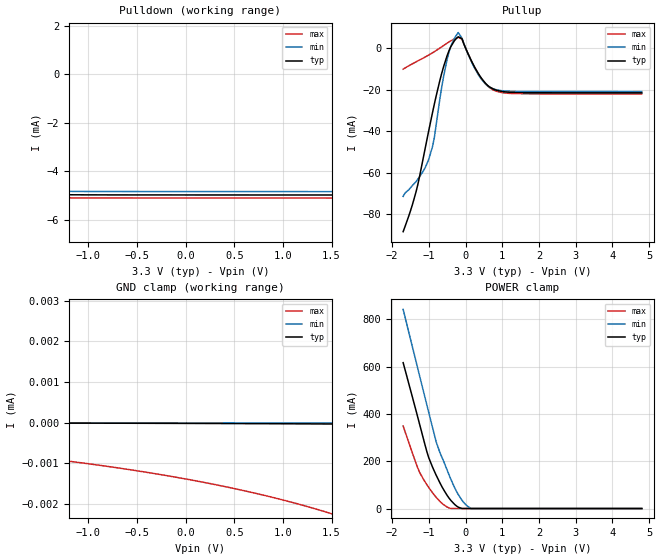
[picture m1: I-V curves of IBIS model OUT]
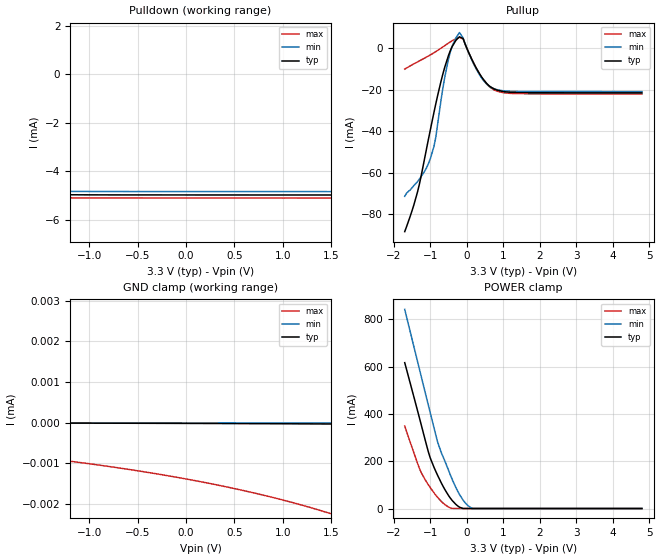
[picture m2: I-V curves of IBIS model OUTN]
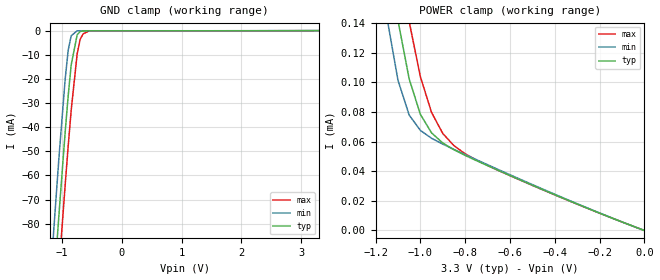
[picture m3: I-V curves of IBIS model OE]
| IBIS File ea2102.ibs
[IBIS Ver]   3.2
[File name]   ea2102.ibs
[File Rev]   1.1
[Date]   April 07,2008
[Disclaimer]
Epson Toyocom Corporation makes no warranty with respect to the information
contained herein.
[Copyright]
Copyright(C) 2008, Epson Toyocom Corporation. All rights reserved.
|   Component EA-2102CB
[Component]   EA-2102CB
Si_location Pin
Timing_location Pin
[Manufacturer]   Epson Toyocom Corporation
[Package]
| variable   typ   min   max
R_pkg   1.04   NA   NA
L_pkg   1.98n   NA   NA
C_pkg   3.71p   NA   NA
[Pin] signal_name   model_name
1   OE   OE
3   GND   GND
4   OUT   OUT
5   OUTN   OUTN
6   VCC   POWER
| Models and submodels in the file (3): OUT (3-state_ECL), OUTN (3-state_ECL), OE (Input)
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|   Model OUT
[Model]   OUT
Model_type 3-state_ECL
Enable Active-High
Polarity Non-Inverting
Vref=1.3
Vmeas=1.97
Rref=50
C_comp   3p   NA   NA
[Temperature Range] 25   -40   85
[Voltage Range]   3.3   3   3.6
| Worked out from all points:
|   GND clamp passes 1 mA (typ) near -3.42 V on its own axis
|   POWER clamp passes 1 mA (typ) near -0.12 V on its own axis
[Pullup]
-1.7V     -88.4mA    -71.42mA   -10.14mA
-1.35V    -69.31mA   -64.36mA   -6.662mA
-1V       -39.54mA   -53.37mA   -3.319mA
-850mV    -26.97mA   -43.09mA   -1.734mA
-650mV    -12.19mA   -18.88mA   598.7uA
-500mV    -3.531mA   -5.232mA   2.399mA
-400mV    718.1uA    1.011mA    3.511mA
-200mV    5.42mA     7.472mA    5.095mA
-100mV    4.565mA    4.85mA     4.38mA
350mV     -12.37mA   -12.87mA   -12.43mA
800mV     -20.07mA   -19.88mA   -20.56mA
4.8V      -21.56mA   -20.96mA   -22.11mA
[Pulldown]
-5V       -23.85mA   -20.89mA   -6.093mA
-4.35V    -14.27mA   -18.44mA   -4.063mA
-3.95V    -6.468mA   -15.25mA   -1.174mA
-3.75V    -3.048mA   -10.1mA    1.119mA
-3.7V     -2.251mA   -8.541mA   1.051mA
-3.6V     -714.4uA   -5.714mA   -1.09nA
-3.5V     888.6uA    -3.303mA   -953.3uA
-3.4V     1.098mA    -1.336mA   -1.821mA
-3.15V    -1.401mA   1.865mA    -3.569mA
-2.7V     -4.216mA   -2.707mA   -4.892mA
-2.25V    -4.871mA   -4.555mA   -5.062mA
1.5V      -4.978mA   -4.838mA   -5.103mA
[GND Clamp]
-5V       616.4mA    841.5mA    348.7mA
-3.7V     34.04mA    123.3mA    185.8uA
-3.6V     17.65mA    88.89mA    326.2fA
-3.55V    11.15mA    73.48mA    -342.5nA
-3.4V     15.09uA    35.4mA     -436.6nA
-3.35V    73.91nA    25.63mA    -447.3nA
-3.3V     0A         17.29mA    -457.5nA
-3.15V    -5.195nA   189.1uA    -487.1nA
-3.1V     -5.365nA   95.47nA    -496.9nA
-3.05V    -5.521nA   147.6pA    -506.6nA
-400mV    -16.4nA    -28.83pA   -1.224uA
1.5V      -33.73nA   -58.18pA   -2.243uA
[POWER Clamp]
-1.7V     616.4mA    841.5mA    348.7mA
-1.35V    414.1mA    622mA      191.6mA
-1.25V    355.1mA    559.5mA    152.4mA
-1.05V    238mA      435.1mA    99.88mA
-900mV    175.1mA    342.6mA    66.68mA
-800mV    140.6mA    281.5mA    47.18mA
-700mV    108.9mA    237mA      30.3mA
-400mV    34.04mA    123.3mA    185.8uA
-200mV    5.735mA    59.39mA    -406.9nA
50mV      -4.322nA   10.2mA     -467.5nA
200mV     -5.365nA   95.47nA    -496.9nA
4.8V      -33.73nA   -58.18pA   -2.243uA
[Ramp]
R_load=50
dV/dt_r   4.714E-1/5.411E-11   4.388E-1/5.767E-11   4.955E-1/5.468E-11
dV/dt_f   4.740E-1/5.706E-11   4.381E-1/6.433E-11   5.010E-1/5.109E-11
| End [model] OUT
|   Model OUTN
[Model]   OUTN
Model_type 3-state_ECL
Enable Active-High
Polarity Inverting
Vref=1.3
Vmeas=1.97
Rref=50
C_comp   3p   NA   NA
[Temperature Range] 25   -40   85
[Voltage Range]   3.3   3   3.6
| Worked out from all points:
|   GND clamp passes 1 mA (typ) near -3.42 V on its own axis
|   POWER clamp passes 1 mA (typ) near -0.12 V on its own axis
[Pullup]
-1.7V     -88.4mA    -71.42mA   -10.14mA
-1.35V    -69.31mA   -64.36mA   -6.662mA
-1V       -39.54mA   -53.37mA   -3.319mA
-850mV    -26.97mA   -43.09mA   -1.734mA
-650mV    -12.19mA   -18.88mA   598.7uA
-500mV    -3.531mA   -5.232mA   2.399mA
-400mV    718.1uA    1.011mA    3.511mA
-200mV    5.42mA     7.472mA    5.095mA
-100mV    4.565mA    4.85mA     4.38mA
350mV     -12.37mA   -12.87mA   -12.43mA
800mV     -20.07mA   -19.88mA   -20.56mA
4.8V      -21.56mA   -20.96mA   -22.11mA
[Pulldown]
-5V       -23.85mA   -20.89mA   -6.093mA
-4.35V    -14.27mA   -18.44mA   -4.063mA
-3.95V    -6.468mA   -15.25mA   -1.174mA
-3.75V    -3.048mA   -10.1mA    1.119mA
-3.7V     -2.251mA   -8.541mA   1.051mA
-3.6V     -714.4uA   -5.714mA   -1.09nA
-3.5V     888.6uA    -3.303mA   -953.3uA
-3.4V     1.098mA    -1.336mA   -1.821mA
-3.15V    -1.401mA   1.865mA    -3.569mA
-2.7V     -4.216mA   -2.707mA   -4.892mA
-2.25V    -4.871mA   -4.555mA   -5.062mA
1.5V      -4.978mA   -4.838mA   -5.103mA
[GND Clamp]
-5V       616.4mA    841.5mA    348.7mA
-3.7V     34.04mA    123.3mA    185.8uA
-3.6V     17.65mA    88.89mA    326.2fA
-3.55V    11.15mA    73.48mA    -342.5nA
-3.4V     15.09uA    35.4mA     -436.6nA
-3.35V    73.91nA    25.63mA    -447.3nA
-3.3V     0A         17.29mA    -457.5nA
-3.15V    -5.195nA   189.1uA    -487.1nA
-3.1V     -5.365nA   95.47nA    -496.9nA
-3.05V    -5.521nA   147.6pA    -506.6nA
-400mV    -16.4nA    -28.83pA   -1.224uA
1.5V      -33.73nA   -58.18pA   -2.243uA
[POWER Clamp]
-1.7V     616.4mA    841.5mA    348.7mA
-1.35V    414.1mA    622mA      191.6mA
-1.25V    355.1mA    559.5mA    152.4mA
-1.05V    238mA      435.1mA    99.88mA
-900mV    175.1mA    342.6mA    66.68mA
-800mV    140.6mA    281.5mA    47.18mA
-700mV    108.9mA    237mA      30.3mA
-400mV    34.04mA    123.3mA    185.8uA
-200mV    5.735mA    59.39mA    -406.9nA
50mV      -4.322nA   10.2mA     -467.5nA
200mV     -5.365nA   95.47nA    -496.9nA
4.8V      -33.73nA   -58.18pA   -2.243uA
[Ramp]
R_load=50
dV/dt_r   4.716E-1/1.034E-10   4.386E-1/1.067E-10   4.953E-1/9.525E-11
dV/dt_f   4.738E-1/6.119E-11   4.380E-1/6.836E-11   5.009E-1/5.282E-11
| End [model] OUTN
|   Model OE
[Model]   OE
Model_type Input
Vinh=2.31
Vinl=0.99
C_comp   3p   3p   3p
[Temperature Range] 25   -40   85
[Voltage Range]   3.3   3   3.6
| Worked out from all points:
|   GND clamp passes 1 mA (typ) near -0.72 V on its own axis
|   POWER clamp passes 1 mA (typ) near -1.64 V on its own axis
[GND Clamp]
-3.3V     -919.3mA   -898.3mA   -939.8mA
-1.15V    -109.5mA   -85.68mA   -132.3mA
-1.1V     -91.92mA   -68.15mA   -114.7mA
-1.05V    -74.68mA   -51.09mA   -97.29mA
-950mV    -41.84mA   -19.94mA   -63.72mA
-900mV    -26.97mA   -8.112mA   -47.85mA
-850mV    -14.25mA   -2.135mA   -33.02mA
-750mV    -1.706mA   -73.58uA   -9.66mA
-700mV    -343.6uA   -56.53uA   -3.634mA
-650mV    -108.1uA   -55.1uA    -1.329mA
-550mV    -69.46uA   -54.93uA   -134.1uA
3.3V      3.304pA    18.04uA    -15.97uA
[POWER Clamp]
-3.3V     4.199mA    4.175mA    4.232mA
-1.15V    195.7uA    144.1uA    250.9uA
-1.1V     141.6uA    101.3uA    190.7uA
-1.05V    102.2uA    77.83uA    140.8uA
-1V       78.31uA    67.5uA     103.7uA
-950mV    65.8uA     62.17uA    79.56uA
-900mV    58.99uA    58.24uA    65.42uA
-850mV    54.42uA    54.67uA    57.15uA
-750mV    47.13uA    47.75uA    47.51uA
-600mV    37.07uA    37.59uA    36.98uA
-300mV    17.83uA    18.04uA    17.75uA
0V        3.297pA    2.995pA    4.576pA
